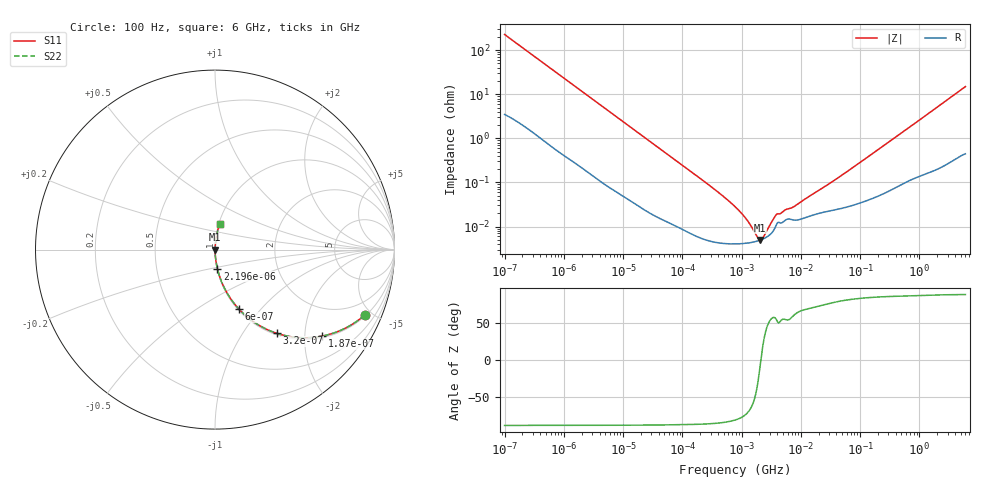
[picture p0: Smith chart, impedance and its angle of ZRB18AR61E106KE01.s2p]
!Murata Part Number: ZRB18AR61E106KE01
!These Parameters are Measured in Series Mode Connection
!Data Generated on Jun 10, 2025
!  o--ll--o
!Port1  Port2
!  o------o
!Operation Temp=25[degC], DC Bias Voltage=0[V]
!Freq. Start=100[Hz] Stop=6[GHz] 401[Steps]
# Hz S RI R 50
!Freq.(Hz) S11(Real) S11(Imag) S21(Real) S21(Imag) S12(Real) S12(Imag) S22(Real) S22(Imag)
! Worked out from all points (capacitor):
!   401 points, 100 Hz to 6 GHz, reference 50 ohm
!   read as one part in series: C = 6.99 uF near 109 Hz
!   lowest |Z| = 4.96 mohm at 2.074 MHz (marker M1)
!   series resonance near 2.123 MHz, so ESL is about 800 pH
!   S11 on the Smith chart (normalised r, x): 100 Hz: 1.07, -4.53; 187 Hz: 1.04, -2.44; 320 Hz: 1.03, -1.44; 600 Hz: 1.01, -0.77; 2.196 kHz: 1.00, -0.21; 6 GHz: 1.01, +0.30
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100  0.8334 -0.365  0.1666 0.365  0.1666 0.365  0.8334 -0.365
187  0.597 -0.4819  0.403 0.4819  0.403 0.4819  0.597 -0.4819
320  0.3431 -0.466  0.6569 0.466  0.6569 0.466  0.3431 -0.466
600  0.1343 -0.3324  0.8657 0.3324  0.8657 0.3324  0.1343 -0.3324
981  0.0569 -0.223  0.9431 0.223  0.9431 0.223  0.0569 -0.223
2008  0.0155 -0.1149  0.9845 0.1149  0.9845 0.1149  0.0155 -0.1149
2196  0.0132 -0.1054  0.9868 0.1054  0.9868 0.1054  0.0132 -0.1054
6728  0.00193 -0.0353  0.9981 0.0353  0.9981 0.0353  0.00193 -0.0353
40335  0.000192 -0.00603  0.9998 0.00603  0.9998 0.00603  0.000192 -0.00603
302498  4.67e-05 -0.000809  1 0.000809  1 0.000809  4.67e-05 -0.000809
774597  4.04e-05 -0.00028  1 0.00028  1 0.00028  4.04e-05 -0.00028
1449809  4.34e-05 -9.24e-05  1 9.24e-05  1 9.24e-05  4.34e-05 -9.24e-05
1585629  4.44e-05 -7.01e-05  1 7.01e-05  1 7.01e-05  4.44e-05 -7.01e-05
2074311  4.93e-05 -5.5e-06  1 5.5e-06  1 5.5e-06  4.93e-05 -5.5e-06
2837864  6.13e-05 7.12e-05  0.9999 -7.12e-05  0.9999 -7.12e-05  6.13e-05 7.12e-05
3882480  0.00011 0.000152  0.9999 -0.000152  0.9999 -0.000152  0.00011 0.000152
7599586  0.00014 0.000243  0.9999 -0.000243  0.9999 -0.000243  0.00014 0.000243
1.555665e7  0.000179 0.000502  0.9998 -0.000502  0.9998 -0.000502  0.000179 0.000502
4.556224e7  0.000254 0.00133  0.9997 -0.00133  0.9997 -0.00133  0.000254 0.00133
3.124326e8  0.000713 0.00841  0.9993 -0.00841  0.9993 -0.00841  0.000713 0.00841
1.791126e9  0.00391 0.0453  0.9961 -0.0453  0.9961 -0.0453  0.00391 0.0453
6e9  0.0258 0.1444  0.9742 -0.1444  0.9742 -0.1444  0.0258 0.1444
